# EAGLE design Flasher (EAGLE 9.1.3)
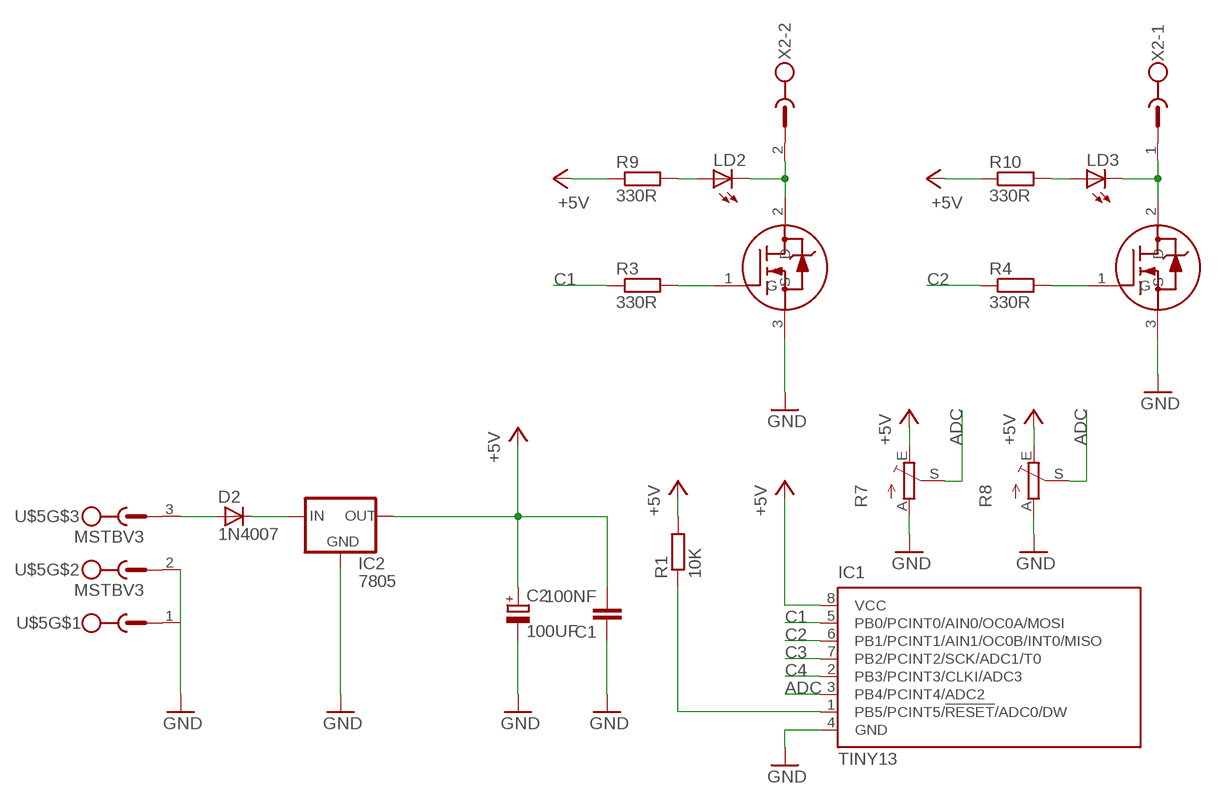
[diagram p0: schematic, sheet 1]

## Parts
C1  100NF  C-EU050-024X044  [C050-024X044]
C2  100UF  CPOL-EUE2.5-5  [E2,5-5]
D2  1N4007  [SMA]
IC1  TINY13  TINY13-20PU  [DIL08]
IC2  7805  78XXS  [78XXS]
LD2  LED5MM  [LED5MM]
LD3  LED5MM  [LED5MM]
R1  10K  R-EU_0204/7  [0204/7]
R3  330R  R-EU_0207/10  [0207/10]
R4  330R  R-EU_0207/10  [0207/10]
R7  TRIM_EU-B25U  [B25U]
R8  TRIM_EU-B25P  [B25P]
R9  330R  R-EU_0204/2V  [0204V]
R10  330R  R-EU_0204/2V  [0204V]
U$1  20N03  [DPAK]
U$3  20N03  [DPAK]
U$5  MSTBV3  [MSTBV3]
X2  MSTBV2  [MSTBV2]

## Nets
+5V: C1.2 C2.+ IC1.8(VCC) IC2.OUT R1.2 R7.E R8.E R9.1 R10.1
ADC: IC1.3(PB4/PCINT4/ADC2) R7.S R8.S
C1: IC1.5(PB0/PCINT0/AIN0/OC0A/MOSI) R3.1
C2: IC1.6(PB1/PCINT1/AIN1/OC0B/INT0/MISO) R4.1
C3: IC1.7(PB2/PCINT2/SCK/ADC1/T0)
C4: IC1.2(PB3/PCINT3/CLKI/ADC3)
GND: C1.1 C2.- IC1.4(GND) IC2.GND R7.A R8.A U$1.3(S) U$3.3(S) U$5.1 U$5.2
N$1: LD2.K(C) U$1.2(D) X2.2
N$2: D2.A U$5.3
N$3: D2.K(C) IC2.IN
N$5: IC1.1(PB5/PCINT5/!RESET!/ADC0/DW) R1.1
N$6: LD3.K(C) U$3.2(D) X2.1
N$9: R3.2 U$1.1(G)
N$12: R4.2 U$3.1(G)
N$13: LD2.A R9.2
N$14: LD3.A R10.2

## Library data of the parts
C1 = rcl:C-EU: CAPACITOR, European symbol
C2 = rcl:CPOL-EU: POLARIZED CAPACITOR, European symbol
D2 = casovac:1N4007
IC1 = atmel:TINY13: 8-bit AVR Microcontroller with 1K Bytes In-System Programmable Flash Source: http://www.atmel.com/dyn/resources/prod_documents/2535S.pdf; MPN: ATTINY13-20PU; OC_FARNELL: 9171550; OC_NEWARK: 96K6521
IC2 = v-reg:78XXS: VOLTAGE REGULATOR
LD2 LD3 = led:LED: LED
R1 R3 R4 R9 R10 = rcl:R-EU_: RESISTOR, European symbol
R7 R8 = pot:TRIM_EU-: POTENTIOMETER
U$1 U$3 = 20n03:20N03
U$5 = con-phoenix-500:MSTBV3
X2 = con-phoenix-500:MSTBV2: PHOENIX; OC_FARNELL: unknown; OC_NEWARK: unknown

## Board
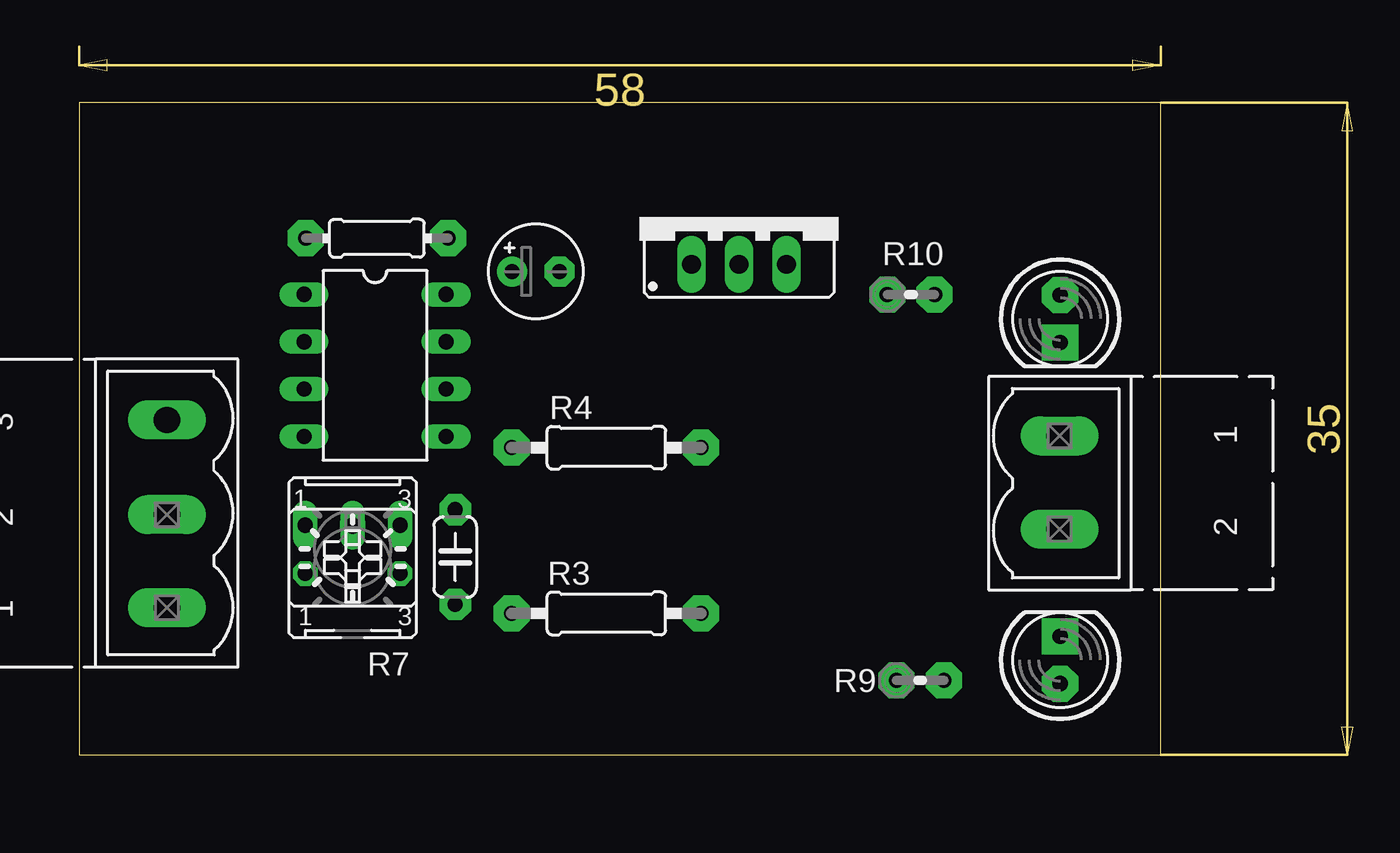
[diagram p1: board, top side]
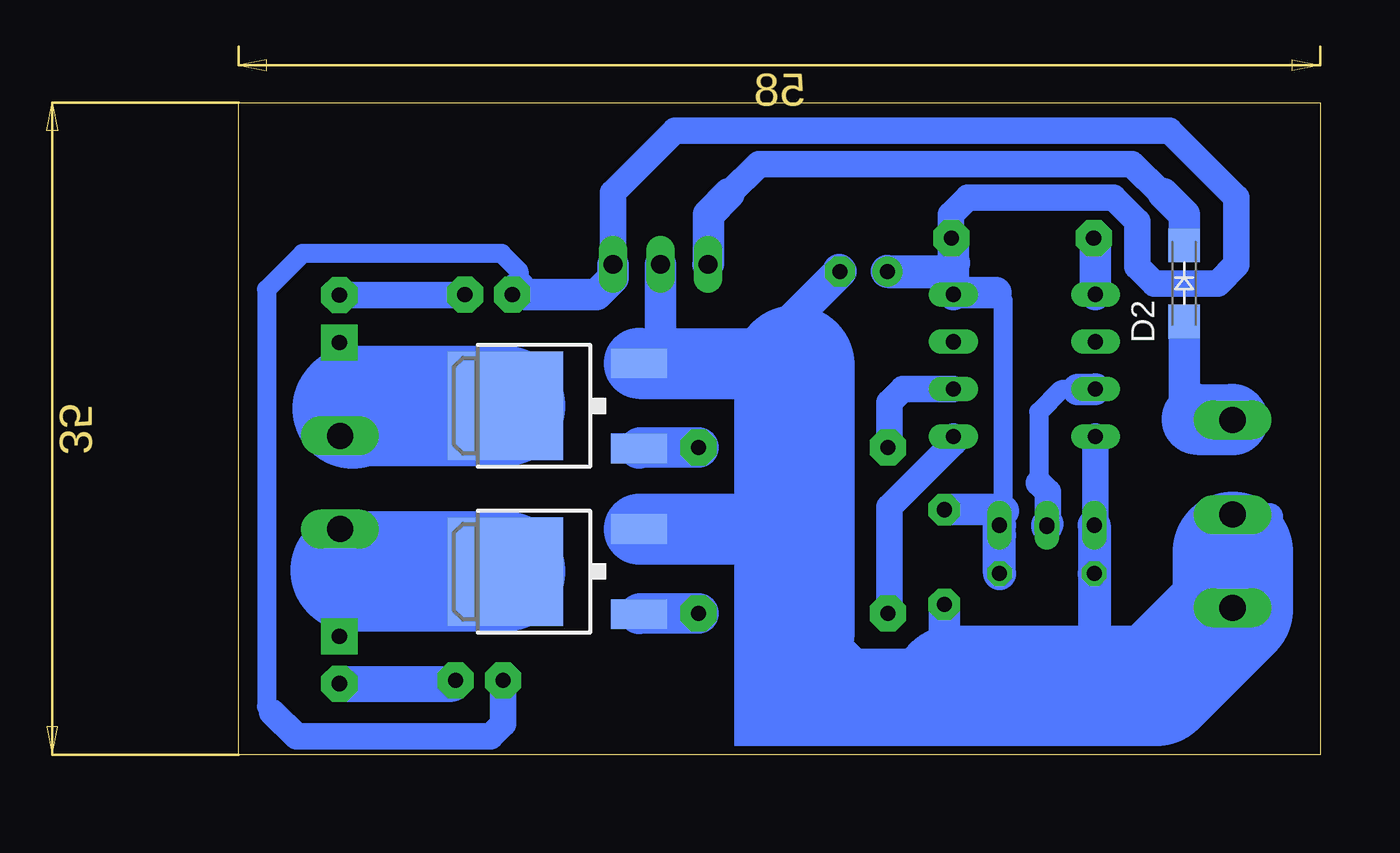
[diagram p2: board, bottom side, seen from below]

Size 68.3 x 38 mm. Coordinates in mm from the lower left corner, seen from the top.
Outline: 0,0 58,0 58,35 0,35 0,0
Copper layers (1*16): Top 0.035mm / dielectric 1.5mm / Bottom 0.035mm
Design rules "default": minimum track width 10mil, minimum drill 24mil, track to track 8mil, track to pad 8mil, pad to pad 8mil, via to via 8mil, smd to smd 8mil, copper to edge 40mil, drill to drill 8mil, minimum pad ring 10mil, minimum via ring 8mil, stop-mask expansion 4mil, vias tented up to drill 0mil, thermal gap 10mil

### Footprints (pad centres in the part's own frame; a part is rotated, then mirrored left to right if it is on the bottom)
C050-024X044 = drill 0.813 pad 1.676 octagon: 1 -2.54,0; 2 2.54,0
E2,5-5 = drill 0.813 pad 1.6: + -1.27,0 | drill 0.813 pad 1.6 octagon: - 1.27,0
SMA = smd 1.8 x 1.7: A -2.05,0; K 2.05,0
DIL08 = drill 0.813 long: 1 -3.81,-3.81; 2 -1.27,-3.81; 3 1.27,-3.81; 4 3.81,-3.81; 5 3.81,3.81; 6 1.27,3.81; 7 -1.27,3.81; 8 -3.81,3.81
78XXS = drill 1.016 long: GND 0,-2.54; IN -2.54,-2.54; OUT 2.54,-2.54
LED5MM = drill 0.813 pad 1.93 octagon: A -1.27,0 | drill 0.813 pad 1.93 square: K 1.27,0
0204/7 = drill 0.813 pad 1.93 octagon: 1 -3.81,0; 2 3.81,0
0207/10 = drill 0.813 pad 1.93 octagon: 1 -5.08,0; 2 5.08,0
B25U = drill 0.813 long: A 2.54,-0.889; E -2.54,-0.889; S 0,-0.889
B25P = drill 0.813 octagon: A -2.54,0; E 2.54,0; S 0,2.54
0204V = drill 0.813 pad 1.93 octagon: 1 -1.27,0; 2 1.27,0
DPAK = smd 1.6 x 3: 1 -2.28,-4.8; 3 2.28,-4.8 | smd 5.8 x 6.2: 2 0,2.38
MSTBV3 = drill 1.397 long: 1 -2.5,0; 2 2.5,0; 3 7.58,0
MSTBV2 = drill 1.397 long: 1 -2.5,0; 2 2.5,0

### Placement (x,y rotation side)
C1  20.16,10.62 90 top
C2  24.48,25.94 0 top
D2  7.3,25.3 90 bottom
IC1  15.86,20.9 270 top
IC2  35.38,28.86 0 top
LD2  52.6,5.1 90 top
LD3  52.6,23.4 270 top
R1  15.96,27.72 0 top
R3  28.27,7.6 0 top
R4  28.27,16.49 0 top
R7  14.66,11.44 180 top
R8  14.66,9.73 0 top
R9  45.1,4 0 top
R10  44.6,24.7 0 top
U$1  41.33,9.84 90 bottom
U$3  41.33,18.73 90 bottom
U$5  4.7,10.4 90 top
X2  52.57,14.62 270 top

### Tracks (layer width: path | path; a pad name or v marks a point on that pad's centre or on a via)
+5V
  Bottom 1.016: 56.2,2.3 56.5,2.6 56.5,24.98 54.58,26.9 43.9,26.9 42.97,25.96 42.97,25.07 | 17.4,24.8 17,24.4 17,13.1 17,12 17.2,11.8
  Bottom 1.422: R9.1 43.83,1.67 44.5,1 54.9,1 56.2,2.3 | IC2.OUT 37.92,30.18 34.6,33.5 8.1,33.5 4.5,29.9 4.5,26.3 5.5,25.3 8.9,25.3 9.8,26.2 9.8,28.6 11.1,29.9 18.9,29.9 19.8,29 19.8,27.75 R1.2
  Bottom 1.676: 17.4,24.8 19.58,24.8 IC1.8 19.67,26.4 19.67,27.62 R1.2 | C1.2 17.06,13.16 17,13.1 | IC2.OUT 37.92,25.58 38.8,24.7 42.6,24.7 42.97,25.07
  Bottom 1.778: R8.E 17.2,11.8 R7.E | C2.+ 20.13,25.94 19.67,26.4 | 42.97,25.07 R10.1
ADC
  Bottom 1.016: 13,19.6 13.9,19.6 15.1,18.4 15.1,14.6
  Bottom 1.422: 14.6,12.39 14.6,14.1 15.1,14.6
  Bottom 1.676: 13,19.6 12.08,19.6 IC1.3 | 14.6,12.39 R7.S R8.S
C1
  Bottom 1.422: IC1.5 19.67,16.73 23.1,13.3 23.1,7.69 R3.1
C2
  Bottom 1.016: 23.1,16.58 R4.1
  Bottom 1.422: IC1.6 22.37,19.63 23.1,18.9 23.1,16.58
GND
  Bottom 1.422: 2.7,12.8 4.6,12.8 U$5.2 | IC1.4 12.05,12.4 R7.A
  Bottom 1.676: C1.1 20.16,3.76 20.1,3.7 | IC2.GND 35.38,21.53 35.9,21.01
  Bottom 1.778: R7.A R8.A 12.12,3.72 12.1,3.7 | 13.12,3.72 13.1,3.7 | 28.2,20.9 28.2,23.49 C2.- 25.8,25.99
  Bottom 2.184: 4.7,10.9 U$5.2
  Bottom 3.81: U$5.1 4.7,7.8 | U$3.3 35.9,21.01 28.81,21.01 28.7,20.9 28.2,20.9 | U$1.3 28.28,12.12 28.2,12.2 | 27.7,6.6 28.2,6.6 25.3,3.7 20.1,3.7 19.7,3.7
  Bottom 6.452: 4.7,7.8 8.8,3.7 12.1,3.7 13.1,3.7 19.7,3.7 | 28.2,6.6 28.2,12.2 28.2,20.9 | U$5.1 4.7,10.9
N$1
  Bottom 1.93: 52,9.9 52,11.55 X2.2 | LD2.K 52.6,9.18 51.94,9.84
  Bottom 6.452: U$1.2 51.94,9.84 52,9.9
N$2
  Bottom 1.676: D2.A 7.3,18.7 6.6,18
  Bottom 3.81: 6.6,18 4.72,18 U$5.3
N$3
  Bottom 1.422: 8.4,30.1 8.5,30.1 10.1,31.7 30.1,31.7 31.7,30.1
  Bottom 1.676: D2.K 7.3,29 8.4,30.1 | 31.7,30.1 32.8,29 32.8,26.36 IC2.IN
N$5
  Bottom 1.676: IC1.1 12.05,27.62 R1.1
N$6
  Bottom 1.778: 51.9,18.6 51.9,18.3 51.9,17.79 X2.1
  Bottom 1.93: LD3.K 52.6,19 51.9,18.3
  Bottom 6.452: U$3.2 51.77,18.73 51.9,18.6
N$9
  Bottom 2.184: R3.2 36.49,7.6 U$1.1
N$12
  Bottom 2.184: R4.2 36.49,16.49 U$3.1
N$13
  Bottom 1.93: LD2.A 46.54,3.83 R9.2
N$14
  Bottom 1.422: LD3.A 45.9,24.67 R10.2
(copper drawn outside any net)
  shapes: Bottom area x2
